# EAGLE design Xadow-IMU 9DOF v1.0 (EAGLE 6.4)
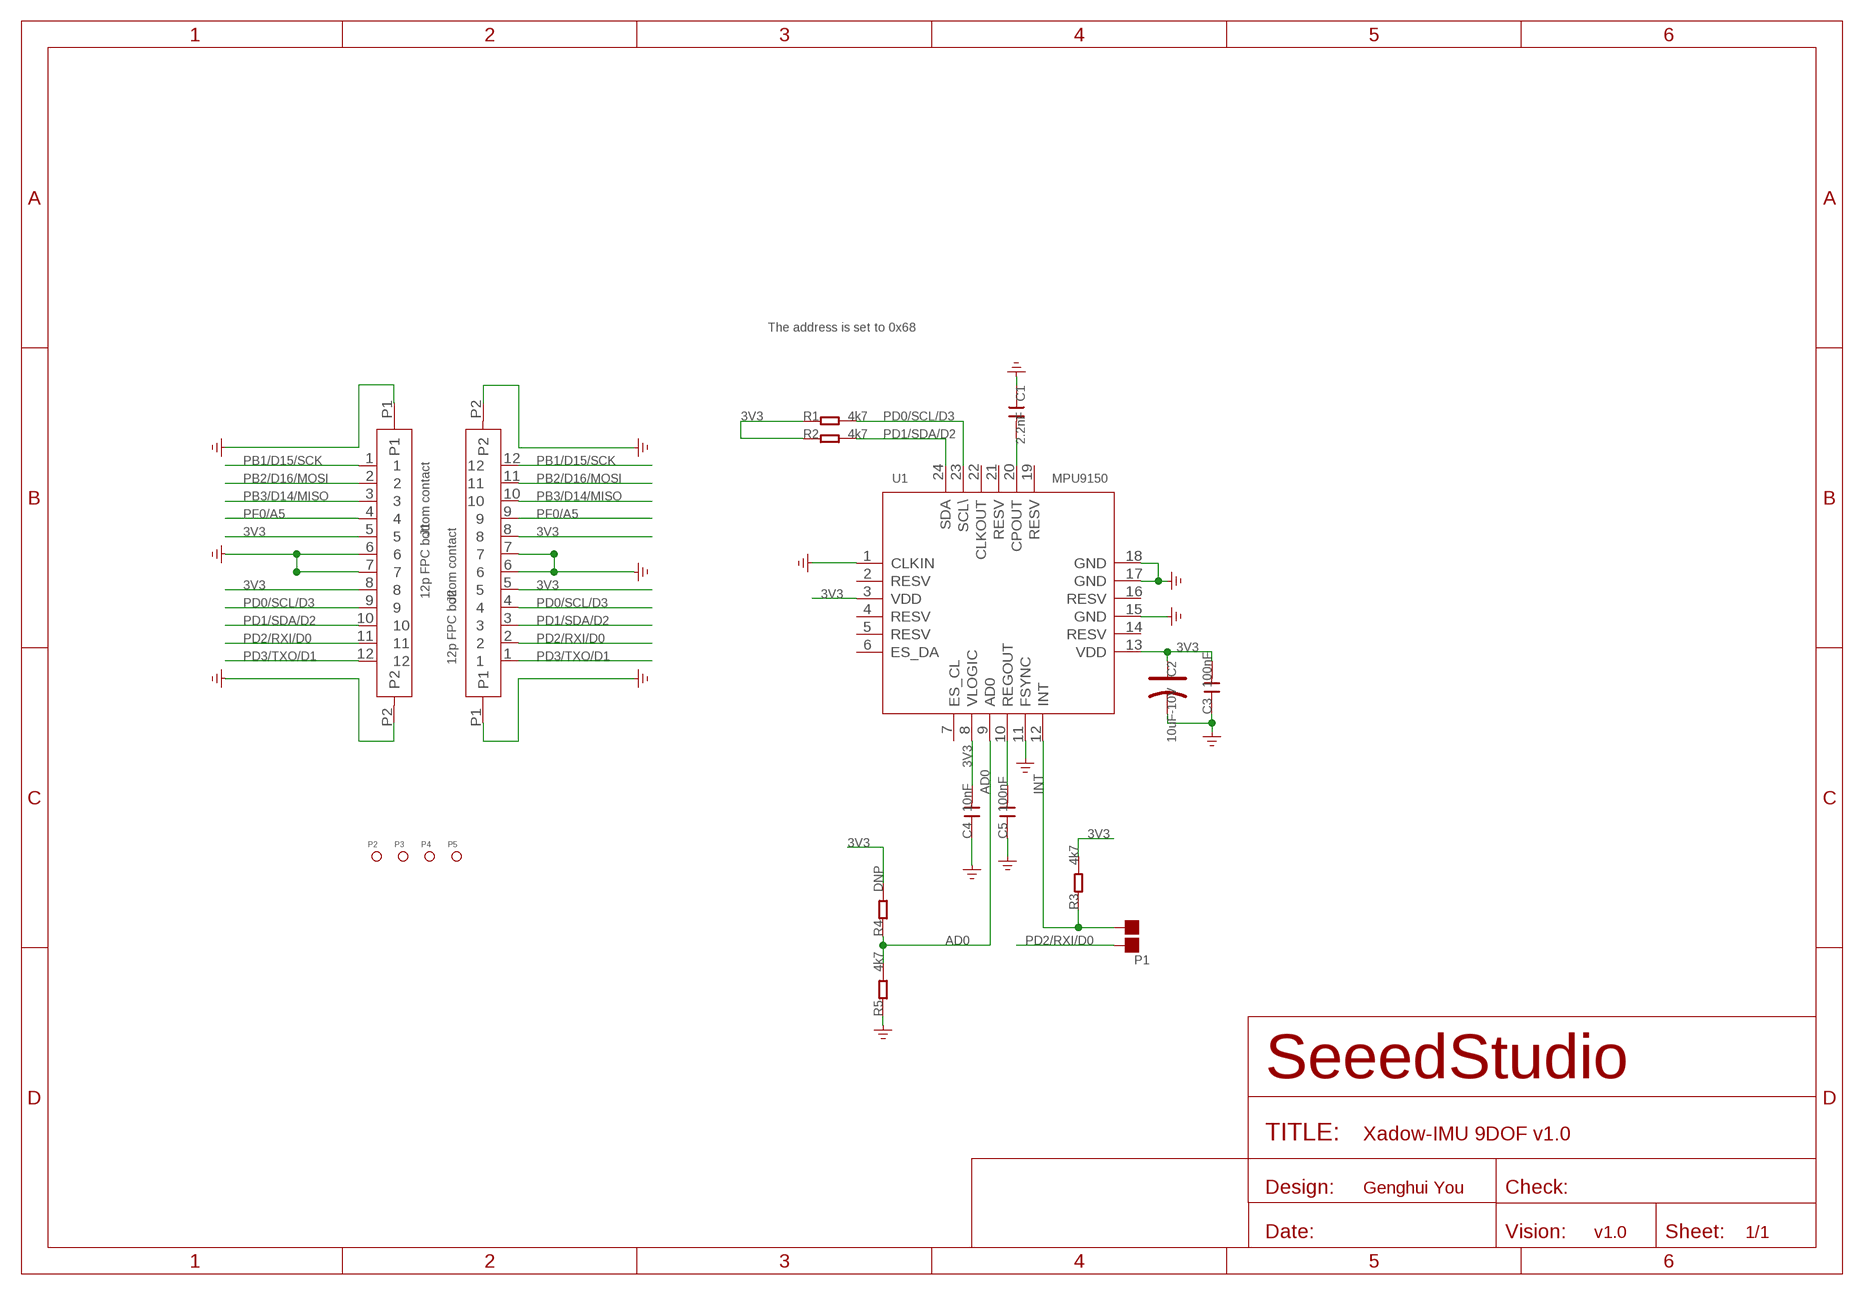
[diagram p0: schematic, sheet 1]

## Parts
C1  2.2nF  C-0603  [C0603]
C2  10uF-10V  CAP-AVX-A  [AVX-A]
C3  100nF  C-0603  [C0603]
C4  10nF  C-0603  [C0603]
C5  100nF  C-0603  [C0603]
J1  12p FPC bottom contact  FPC052002-12LT  [12P-0.5-NEW]
J2  12p FPC bottom contact  FPC052002-12LT  [12P-0.5-NEW]
P1  PAD-JUMPER-2P  [2P-SMD-1.78X1.27]
P2  PAD-MARK  [ROUND-MARK-1.0]
P3  PAD-MARK  [ROUND-MARK-1.0]
P4  PAD-MARK  [ROUND-MARK-1.0]
P5  PAD-MARK  [ROUND-MARK-1.0]
R1  4k7  R-0603  [R0603]
R2  4k7  R-0603  [R0603]
R3  4k7  R-0603  [R0603]
R4  DNP  R-0603  [R0603]
R5  4k7  R-0603  [R0603]
U1  MPU9150  MPU-9150  [LGA-24]

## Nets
3V3: C2.+ C3.2 C4.2 J1.5 J1.8 J2.5 J2.8 R1.1 R2.1 R3.2 R4.2 U1.3(VDD) U1.8(VLOGIC) U1.13(VDD)
AD0: R4.1 R5.2 U1.9(AD0)
GND: C1.1 C2.- C3.1 C4.1 C5.1 J1.6 J1.7 J1.P1 J1.P2 J2.6 J2.7 J2.P1 J2.P2 R5.1 U1.1(CLKIN) U1.11(FSYNC) U1.15(GND) U1.17(GND) U1.18(GND)
INT: P1.1 R3.1 U1.12(INT)
N$2: C1.2 U1.20(CPOUT)
N$5: C5.2 U1.10(REGOUT)
PB1/D15/SCK: J1.1 J2.12
PB2/D16/MOSI: J1.2 J2.11
PB3/D14/MISO: J1.3 J2.10
PD0/SCL/D3: J1.9 J2.4 R1.2 U1.23(SCL\)
PD1/SDA/D2: J1.10 J2.3 R2.2 U1.24(SDA)
PD2/RXI/D0: J1.11 J2.2 P1.2
PD3/TXO/D1: J1.12 J2.1
PF0/A5: J1.4 J2.9
Unconnected: U1.2(RESV) U1.4(RESV) U1.5(RESV) U1.6(ES_DA) U1.7(ES_CL) U1.14(RESV) U1.16(RESV) U1.19(RESV) U1.21(RESV) U1.22(CLKOUT)

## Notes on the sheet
- The address is set to 0x68
- Genghui You
- v1.0

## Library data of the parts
C1 C3-C5 = Discrete:C*: Ceramic Capacitors
C2 = Discrete:CAP*: Electrolytic Capacitors,Tantalum Capacitors and Super Capacitors
J1 J2 = template:FPC052002-12LT
P1 = Discrete:PAD-JUMPER-2P; PARTNO: DNP
P2-P5 = Discrete:PAD-MARK; PARTNO: DNP
R1-R5 = Discrete:R*
U1 = template:MPU-9150

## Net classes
0 default: width 0.152 mm, drill 0.305 mm, clearance 0.152 mm
1 GND: width 0.152 mm, drill 0.305 mm, clearance 0.152 mm to class 0, clearance 0.152 mm

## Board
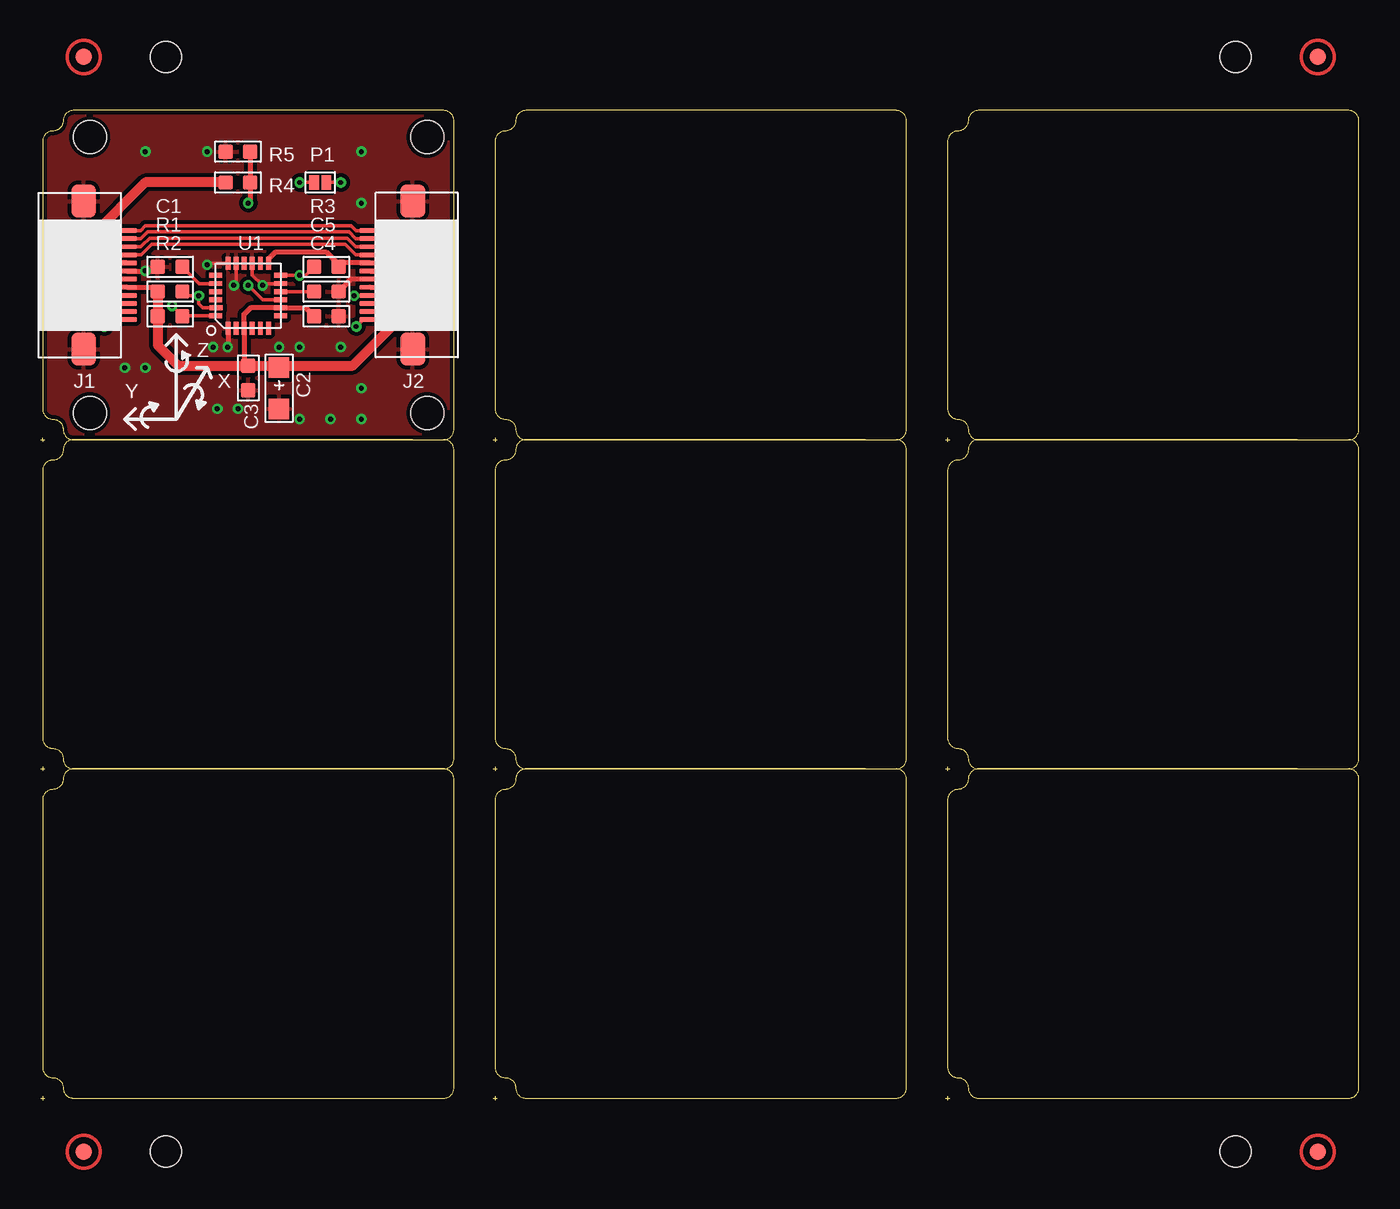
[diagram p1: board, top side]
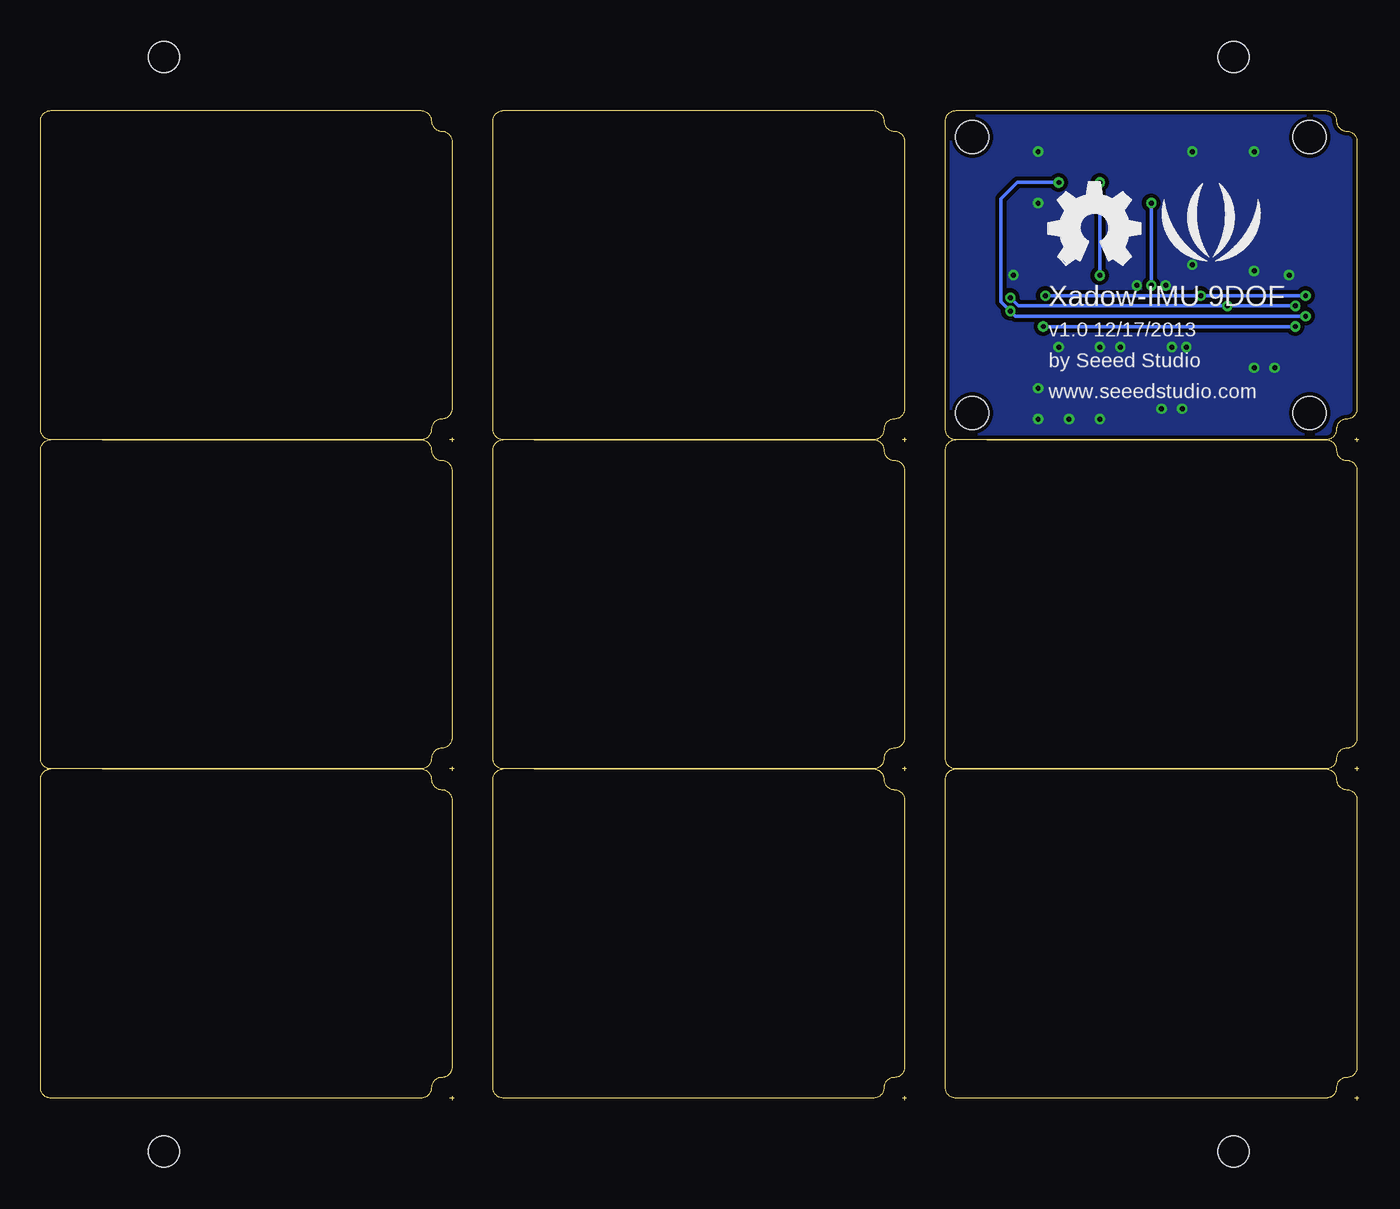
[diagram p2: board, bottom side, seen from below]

Size 81.41 x 61.09 mm. Coordinates in mm from the lower left corner, seen from the top.
Outline: 193 segments
Copper layers (1*16): Top 0.035mm / dielectric 1.5mm / Bottom 0.035mm
Design rules "SeeedStudio_rule_no_angle_090911 *": minimum track width 6mil, minimum drill 12mil, track to track 6mil, track to pad 6mil, pad to pad 6mil, via to via 6mil, smd to smd 0mil, copper to edge 10mil, drill to drill 10mil, minimum pad ring 10mil, minimum via ring 6mil, stop-mask expansion 2mil, vias tented up to drill 100mil, thermal gap 10mil
Holes 2.03 mm at 3.05,42.42 3.05,59.44 23.88,59.44 23.88,42.42
Holes 1.91 mm at 73.79,64.39 7.75,64.39 7.75,-3.17 73.79,-3.17
tRestrict: area 4.6,50.9 to 5.2,51; area 20.4,50.9 to 21,51; area 11.7,51.4 to 11.9,51.9; 13 lines
bRestrict: 13 lines

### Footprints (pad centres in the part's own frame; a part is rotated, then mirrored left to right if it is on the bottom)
C0603 = smd 0.889 x 0.889: 1 -0.762,0; 2 0.762,0
AVX-A = smd 1.27 x 1.27: + -1.27,0; - 1.27,0
12P-0.5-NEW = smd 0.3 x 1.3: 1 -2.75,2.646; 2 -2.25,2.646; 3 -1.75,2.646; 4 -1.25,2.646; 5 -0.75,2.646; 6 -0.25,2.646; 7 0.25,2.646; 8 0.75,2.646; 9 1.25,2.646; 10 1.75,2.646; 11 2.25,2.646; 12 2.75,2.646 | smd 2.032 x 1.524: P1 -4.572,0; P2 4.572,0
2P-SMD-1.78X1.27 = smd 0.889 x 0.61: 1 0,0.381; 2 0,-0.381
ROUND-MARK-1.0 = smd 1.016 x 1.016: P$1 0,0
R0603 = smd 0.889 x 0.889: 1 -0.762,0; 2 0.762,0
LGA-24 = smd 0.8 x 0.3: 1 -2,1.25; 2 -2,0.75; 3 -2,0.25; 4 -2,-0.25; 5 -2,-0.75; 6 -2,-1.25; 13 2,-1.25; 14 2,-0.75; 15 2,-0.25; 16 2,0.25; 17 2,0.75; 18 2,1.25 | smd 0.3 x 0.8: 7 -1.25,-2; 8 -0.75,-2; 9 -0.25,-2; 10 0.25,-2; 11 0.75,-2; 12 1.25,-2; 19 1.25,2; 20 0.75,2; 21 0.25,2; 22 -0.25,2; 23 -0.75,1.975; 24 -1.25,2

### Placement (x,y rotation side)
C1  8,51.44 0 top
C2  14.73,43.94 270 top
C3  12.83,44.58 90 top
C4  17.65,48.39 180 top
C5  17.65,49.91 180 top
J1  2.67,50.93 270 top
J2  22.99,50.93 90 top
P1  17.27,56.64 90 top
P2  not placed on the board
P3  not placed on the board
P4  not placed on the board
P5  not placed on the board
R1  8,49.91 0 top
R2  8,48.39 0 top
R3  17.65,51.44 0 top
R4  12.19,56.64 180 top
R5  12.19,58.55 0 top
U1  12.83,49.66 90 top
U$2  [LOGO_SILK]  9.14,53.47 0 bottom
U$3  [OSHW_FILLX200_NOTEXT]  19.18,51.56 0 bottom

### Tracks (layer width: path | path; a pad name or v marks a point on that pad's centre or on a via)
3V3
  Top 0.203: C2.+ 14.73,45.34
  Top 0.305: C4.2 16.37,48.91 U1.8 12.97,48.91 12.58,48.52 | 12.58,48.52 12.57,48.51 | 12.58,48.52 U1.3 12.58,45.59 C3.2 | 18.41,51.56 R3.2 18.66,51.68 | 18.66,51.68 J2.8 21.6,51.68 22.35,50.93 | J2.5 21.96,50.18 | 21.98,50.18 22.21,50.18 22.35,50.04 | 18.66,51.68 18.3,51.68 17.65,52.32 14.48,52.32 14.08,51.92 U1.13 | 21.96,50.18 21.98,50.18 | 21.98,50.18 22.23,50.42 22.23,49.91 21.96,50.18 | R1.1 6.97,50.18 J1.8 4.05,50.18 3.3,50.93 | J1.5 3.7,51.68 | 3.67,51.68 3.31,51.68 3.3,51.69 | 3.7,51.68 3.43,51.94 3.43,51.44 3.67,51.68 | 3.7,51.68 3.67,51.68
  Top 0.61: 14.73,45.34 19.28,45.34 22.35,48.41 22.35,50.04 22.35,50.93 | C2.+ 14.61,45.34 C3.2 8.51,45.34 7.24,46.61 R2.1 R1.1 | 3.3,50.93 3.3,51.69 3.3,53.47 6.48,56.64 R4.2
AD0  (via drill 0.3 pad 0.64)
  Top 0.203: U1.9 13.71,49.41 v12.83,50.29
  Top 0.305: R5.2 R4.1 12.95,55.5 v12.83,55.37
  Bottom 0.203: v12.83,50.29 v12.83,55.37
GND  (via drill 0.3 pad 0.64)
  Top 0.203: U1.11 13.83,50.41 v13.72,50.29 13.08,50.93 U1.15 | U1.17 12.08,50.43 v11.94,50.29 | U1.18 10.38,51.66 v10.29,51.56
  Top 0.305: C5.1 19.18,50.68 J2.6 21.34,50.67 21.46,50.8 21.46,51.05 21.34,51.18 J2.7 | C1.1 6.98,51.18 J1.6 4.45,51.18 4.32,51.05 4.32,50.8 4.44,50.68 J1.7 | U1.1 11.58,46.5 v11.56,46.48
  other vias: 18.54,46.48 16,46.48 10.67,46.48 16,42.04 12.19,42.67 10.92,42.67 17.91,42.04 6.48,58.55 10.29,58.55 19.81,58.55 5.21,45.21 6.48,45.21 19.81,55.37 19.81,43.94 19.81,42.04 14.73,46.48 6.48,51.18 4.32,50.93 21.34,50.93
  pour Top (isolate 0.254): 0.13,40.77 25.53,40.77 25.53,61.09 0.13,61.09
  pour Bottom (isolate 0.254): 0.13,40.77 25.53,40.77 25.53,61.09 0.13,61.09
INT  (via drill 0.3 pad 0.64)
  Top 0.203: U1.12 v16,50.91 16.36,50.91 R3.1 | P1.1 v16,56.64
  Bottom 0.203: v16,50.91 v16,56.64
N$2
  Top 0.203: U1.20 9.79,50.41 C1.2
N$5
  Top 0.203: U1.10 C5.2
PB1/D15/SCK
  Top 0.203: J2.12 19.48,53.68 19.18,53.98 6.48,53.98 6.18,53.68 J1.1
PB2/D16/MOSI
  Top 0.203: J2.11 19.47,53.18 19.05,53.59 6.6,53.59 6.19,53.18 J1.2
PB3/D14/MISO
  Top 0.203: J2.10 19.46,52.68 18.92,53.21 6.73,53.21 6.29,52.77 6.22,52.7 6.2,52.68 J1.3
PD0/SCL/D3  (via drill 0.3 pad 0.64)
  Top 0.203: J2.4 19.83,49.68 19.81,49.66 v19.37,49.66 | J1.9 5.33,49.66 v3.3,49.66 | U1.23 10.02,48.91 9.78,49.15 v9.78,49.66 8.89,49.66 | 8.89,49.66 8.76,49.78 R1.2 8.76,49.66 8.89,49.66
  Bottom 0.203: v3.3,49.66 v9.78,49.66 v19.37,49.66
PD1/SDA/D2  (via drill 0.3 pad 0.64)
  Top 0.203: U1.24 8.78,48.41 R2.2 v8.13,49.02 | v3.94,49.02 4.09,49.18 J1.10 | J2.3 21.17,49.18 v21.53,49.53
  Bottom 0.203: v3.94,49.02 v8.13,49.02 21.02,49.02 v21.53,49.53
PD2/RXI/D0  (via drill 0.3 pad 0.64)
  Top 0.203: v3.3,48.39 4.19,48.39 4.48,48.68 J1.11 | J2.2 21.5,48.68 v21.53,48.7 | v18.54,56.64 P1.2
  Bottom 0.203: v3.3,48.39 21.21,48.39 v21.53,48.7 22.1,49.28 22.1,55.63 21.08,56.64 v18.54,56.64
PD3/TXO/D1  (via drill 0.3 pad 0.64)
  Top 0.203: J2.1 19.79,48.18 19.79,48.05 | J1.12 4.49,48.18 4.06,47.75 v3.94,47.75 | 19.79,48.05 v19.5,47.75 | 19.79,48.05 19.88,48.13
  Bottom 0.203: v3.94,47.75 v19.5,47.75
PF0/A5
  Top 0.203: J2.9 19.45,52.18 18.8,52.83 6.86,52.83 6.2,52.18 J1.4

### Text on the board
tPlace: Z | X | Y
bPlace: Xadow-IMU 9DOF | v1.0 12/17/2013 | by Seeed Studio | www.seeedstudio.com
tEnhance: Top Enhance 0.25~0.28mm
bEnhance: Bottom Enhance
bEnHoles: Holes on Bottom Enhance | All Holes are 70mil diameter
